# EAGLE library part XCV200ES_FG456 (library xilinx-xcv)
xcv200es_fg456 edit this description Auto generated by make-symbol-device-package-bsdl.ulp Rev. 26 Source: xcv200es_fg456.bsd
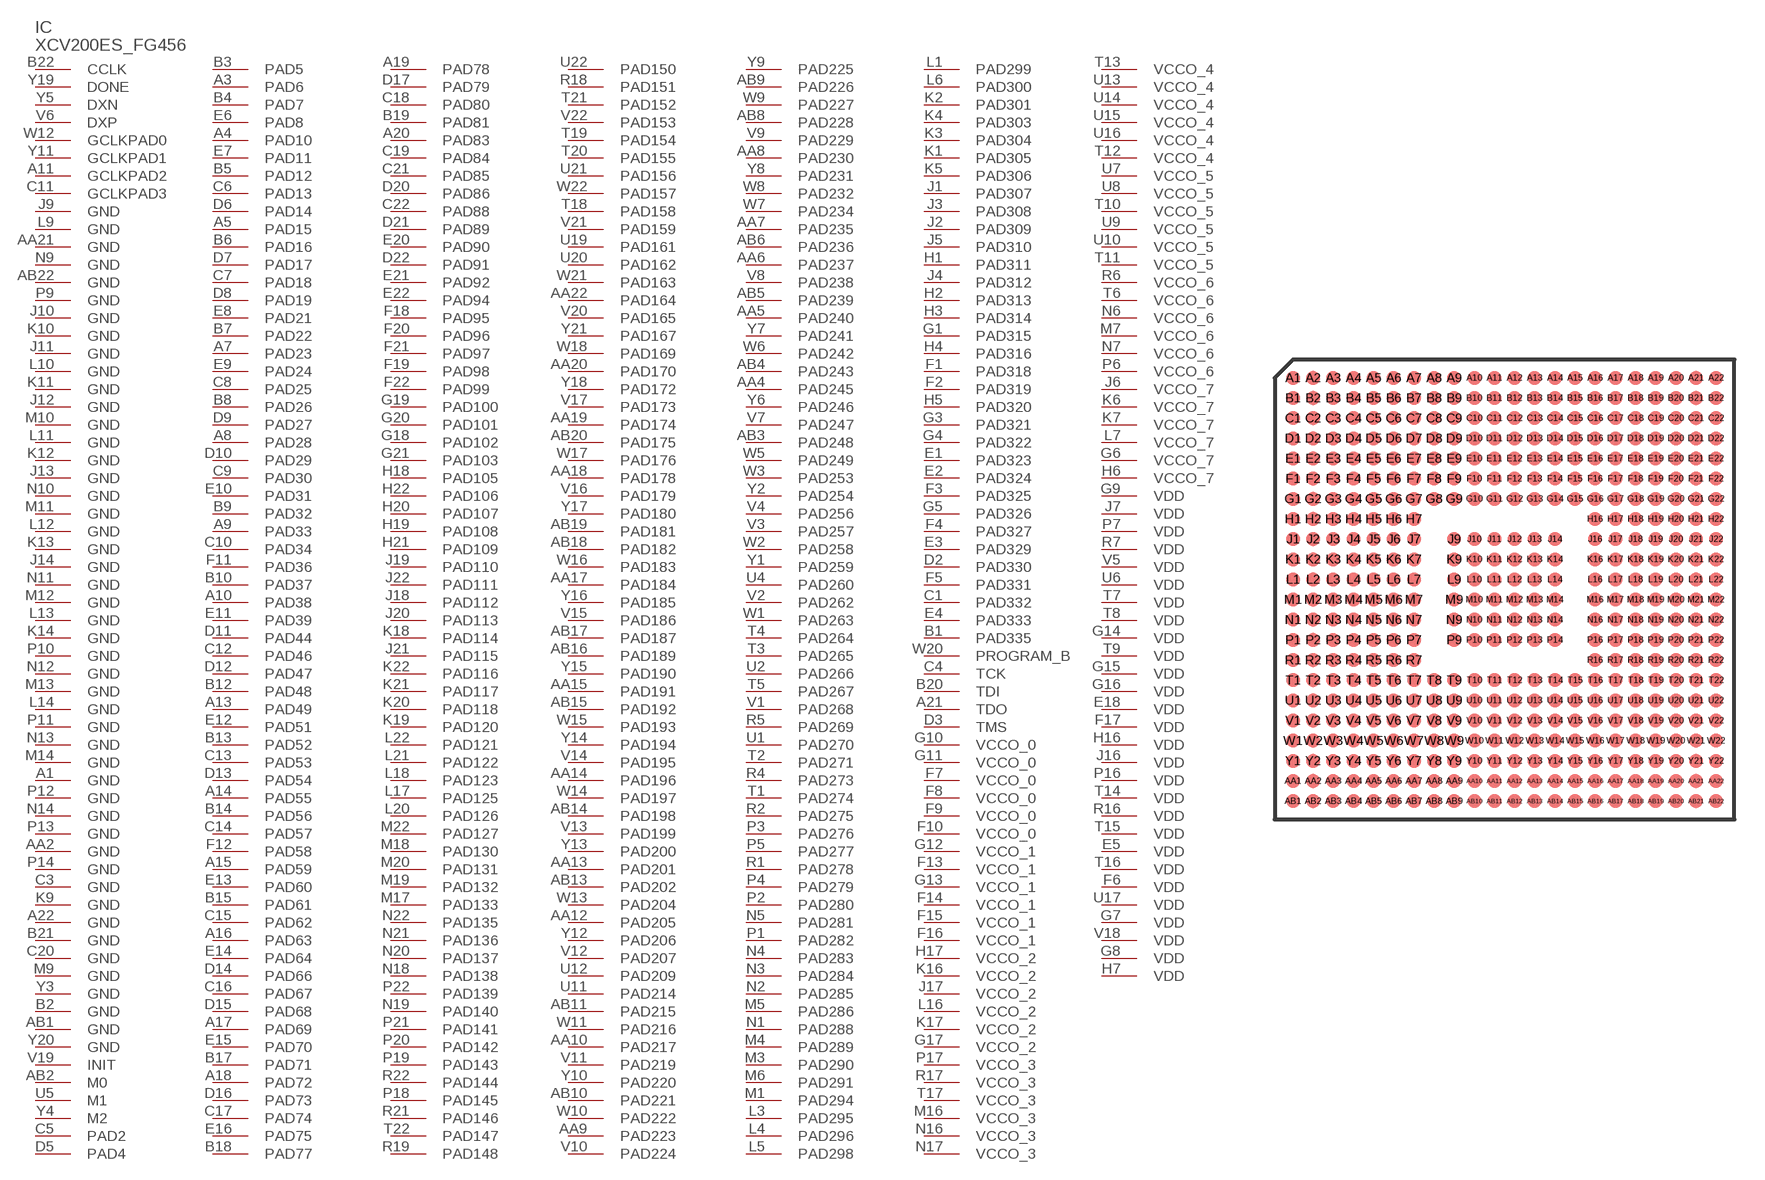
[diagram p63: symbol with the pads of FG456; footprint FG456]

Designator prefix IC

## XCV200ES_FG456 (OC_FARNELL: unknown; OC_NEWARK: unknown)  [FG456]
A1  GND  pwr
A3  PAD6
A4  PAD10
A5  PAD15
A7  PAD23
A8  PAD28
A9  PAD33
A10  PAD38
A11  GCLKPAD2  in
A13  PAD49
A14  PAD55
A15  PAD59
A16  PAD63
A17  PAD69
A18  PAD72
A19  PAD78
A20  PAD83
A21  TDO  out
A22  GND  pwr
AA2  GND  pwr
AA4  PAD245
AA5  PAD240
AA6  PAD237
AA7  PAD235
AA8  PAD230
AA9  PAD223
AA10  PAD217
AA12  PAD205
AA13  PAD201
AA14  PAD196
AA15  PAD191
AA17  PAD184
AA18  PAD178
AA19  PAD174
AA20  PAD170
AA21  GND  pwr
AA22  PAD164
AB1  GND  pwr
AB2  M0  in
AB3  PAD248
AB4  PAD243
AB5  PAD239
AB6  PAD236
AB8  PAD228
AB9  PAD226
AB10  PAD221
AB11  PAD215
AB13  PAD202
AB14  PAD198
AB15  PAD192
AB16  PAD189
AB17  PAD187
AB18  PAD182
AB19  PAD181
AB20  PAD175
AB22  GND  pwr
B1  PAD335
B2  GND  pwr
B3  PAD5
B4  PAD7
B5  PAD12
B6  PAD16
B7  PAD22
B8  PAD26
B9  PAD32
B10  PAD37
B12  PAD48
B13  PAD52
B14  PAD56
B15  PAD61
B17  PAD71
B18  PAD77
B19  PAD81
B20  TDI  in
B21  GND  pwr
B22  CCLK
C1  PAD332
C3  GND  pwr
C4  TCK  in
C5  PAD2
C6  PAD13
C7  PAD18
C8  PAD25
C9  PAD30
C10  PAD34
C11  GCLKPAD3  in
C12  PAD46
C13  PAD53
C14  PAD57
C15  PAD62
C16  PAD67
C17  PAD74
C18  PAD80
C19  PAD84
C20  GND  pwr
C21  PAD85
C22  PAD88
D2  PAD330
D3  TMS  in
D5  PAD4
D6  PAD14
D7  PAD17
D8  PAD19
D9  PAD27
D10  PAD29
D11  PAD44
D12  PAD47
D13  PAD54
D14  PAD66
D15  PAD68
D16  PAD73
D17  PAD79
D20  PAD86
D21  PAD89
D22  PAD91
E1  PAD323
E2  PAD324
E3  PAD329
E4  PAD333
E5  VDD  pwr
E6  PAD8
E7  PAD11
E8  PAD21
E9  PAD24
E10  PAD31
E11  PAD39
E12  PAD51
E13  PAD60
E14  PAD64
E15  PAD70
E16  PAD75
E18  VDD  pwr
E20  PAD90
E21  PAD92
E22  PAD94
F1  PAD318
F2  PAD319
F3  PAD325
F4  PAD327
F5  PAD331
F6  VDD  pwr
F7  VCCO_0  pwr
F8  VCCO_0  pwr
F9  VCCO_0  pwr
F10  VCCO_0  pwr
F11  PAD36
F12  PAD58
F13  VCCO_1  pwr
F14  VCCO_1  pwr
F15  VCCO_1  pwr
F16  VCCO_1  pwr
F17  VDD  pwr
F18  PAD95
F19  PAD98
F20  PAD96
F21  PAD97
F22  PAD99
G1  PAD315
G3  PAD321
G4  PAD322
G5  PAD326
G6  VCCO_7  pwr
G7  VDD  pwr
G8  VDD  pwr
G9  VDD  pwr
G10  VCCO_0  pwr
G11  VCCO_0  pwr
G12  VCCO_1  pwr
G13  VCCO_1  pwr
G14  VDD  pwr
G15  VDD  pwr
G16  VDD  pwr
G17  VCCO_2  pwr
G18  PAD102
G19  PAD100
G20  PAD101
G21  PAD103
H1  PAD311
H2  PAD313
H3  PAD314
H4  PAD316
H5  PAD320
H6  VCCO_7  pwr
H7  VDD  pwr
H16  VDD  pwr
H17  VCCO_2  pwr
H18  PAD105
H19  PAD108
H20  PAD107
H21  PAD109
H22  PAD106
J1  PAD307
J2  PAD309
J3  PAD308
J4  PAD312
J5  PAD310
J6  VCCO_7  pwr
J7  VDD  pwr
J9  GND  pwr
J10  GND  pwr
J11  GND  pwr
J12  GND  pwr
J13  GND  pwr
J14  GND  pwr
J16  VDD  pwr
J17  VCCO_2  pwr
J18  PAD112
J19  PAD110
J20  PAD113
J21  PAD115
J22  PAD111
K1  PAD305
K2  PAD301
K3  PAD304
K4  PAD303
K5  PAD306
K6  VCCO_7  pwr
K7  VCCO_7  pwr
K9  GND  pwr
K10  GND  pwr
K11  GND  pwr
K12  GND  pwr
K13  GND  pwr
K14  GND  pwr
K16  VCCO_2  pwr
K17  VCCO_2  pwr
K18  PAD114
K19  PAD120
K20  PAD118
K21  PAD117
K22  PAD116
L1  PAD299
L3  PAD295
L4  PAD296
L5  PAD298
L6  PAD300
L7  VCCO_7  pwr
L9  GND  pwr
L10  GND  pwr
L11  GND  pwr
L12  GND  pwr
L13  GND  pwr
L14  GND  pwr
L16  VCCO_2  pwr
L17  PAD125
L18  PAD123
L20  PAD126
L21  PAD122
L22  PAD121
M1  PAD294
M3  PAD290
M4  PAD289
M5  PAD286
M6  PAD291
M7  VCCO_6  pwr
M9  GND  pwr
M10  GND  pwr
M11  GND  pwr
M12  GND  pwr
M13  GND  pwr
M14  GND  pwr
M16  VCCO_3  pwr
M17  PAD133
M18  PAD130
M19  PAD132
M20  PAD131
M22  PAD127
N1  PAD288
N2  PAD285
N3  PAD284
N4  PAD283
N5  PAD281
N6  VCCO_6  pwr
N7  VCCO_6  pwr
N9  GND  pwr
N10  GND  pwr
N11  GND  pwr
N12  GND  pwr
N13  GND  pwr
N14  GND  pwr
N16  VCCO_3  pwr
N17  VCCO_3  pwr
N18  PAD138
N19  PAD140
N20  PAD137
N21  PAD136
N22  PAD135
P1  PAD282
P2  PAD280
P3  PAD276
P4  PAD279
P5  PAD277
P6  VCCO_6  pwr
P7  VDD  pwr
P9  GND  pwr
P10  GND  pwr
P11  GND  pwr
P12  GND  pwr
P13  GND  pwr
P14  GND  pwr
P16  VDD  pwr
P17  VCCO_3  pwr
P18  PAD145
P19  PAD143
P20  PAD142
P21  PAD141
P22  PAD139
R1  PAD278
R2  PAD275
R4  PAD273
R5  PAD269
R6  VCCO_6  pwr
R7  VDD  pwr
R16  VDD  pwr
R17  VCCO_3  pwr
R18  PAD151
R19  PAD148
R21  PAD146
R22  PAD144
T1  PAD274
T2  PAD271
T3  PAD265
T4  PAD264
T5  PAD267
T6  VCCO_6  pwr
T7  VDD  pwr
T8  VDD  pwr
T9  VDD  pwr
T10  VCCO_5  pwr
T11  VCCO_5  pwr
T12  VCCO_4  pwr
T13  VCCO_4  pwr
T14  VDD  pwr
T15  VDD  pwr
T16  VDD  pwr
T17  VCCO_3  pwr
T18  PAD158
T19  PAD154
T20  PAD155
T21  PAD152
T22  PAD147
U1  PAD270
U2  PAD266
U4  PAD260
U5  M1  in
U6  VDD  pwr
U7  VCCO_5  pwr
U8  VCCO_5  pwr
U9  VCCO_5  pwr
U10  VCCO_5  pwr
U11  PAD214
U12  PAD209
U13  VCCO_4  pwr
U14  VCCO_4  pwr
U15  VCCO_4  pwr
U16  VCCO_4  pwr
U17  VDD  pwr
U19  PAD161
U20  PAD162
U21  PAD156
U22  PAD150
V1  PAD268
V2  PAD262
V3  PAD257
V4  PAD256
V5  VDD  pwr
V6  DXP  pas
V7  PAD247
V8  PAD238
V9  PAD229
V10  PAD224
V11  PAD219
V12  PAD207
V13  PAD199
V14  PAD195
V15  PAD186
V16  PAD179
V17  PAD173
V18  VDD  pwr
V19  INIT
V20  PAD165
V21  PAD159
V22  PAD153
W1  PAD263
W2  PAD258
W3  PAD253
W5  PAD249
W6  PAD242
W7  PAD234
W8  PAD232
W9  PAD227
W10  PAD222
W11  PAD216
W12  GCLKPAD0  in
W13  PAD204
W14  PAD197
W15  PAD193
W16  PAD183
W17  PAD176
W18  PAD169
W20  PROGRAM_B  in
W21  PAD163
W22  PAD157
Y1  PAD259
Y2  PAD254
Y3  GND  pwr
Y4  M2  in
Y5  DXN  pas
Y6  PAD246
Y7  PAD241
Y8  PAD231
Y9  PAD225
Y10  PAD220
Y11  GCLKPAD1  in
Y12  PAD206
Y13  PAD200
Y14  PAD194
Y15  PAD190
Y16  PAD185
Y17  PAD180
Y18  PAD172
Y19  DONE
Y20  GND  pwr
Y21  PAD167

## Footprint FG456 (pad centres in mm)
xcv150_fg456 edit this description Auto generated by make-symbol-device-package-bsdl.ulp Rev. 26 Source: xcv150_fg456.bsd
smd 0.7 x 0.7: A1 -10.5,10.5; A2 -9.5,10.5; A3 -8.5,10.5; A4 -7.5,10.5; A5 -6.5,10.5; A6 -5.5,10.5; A7 -4.5,10.5; A8 -3.5,10.5; A9 -2.5,10.5; A10 -1.5,10.5; A11 -0.5,10.5; A12 0.5,10.5; A13 1.5,10.5; A14 2.5,10.5; A15 3.5,10.5; A16 4.5,10.5; A17 5.5,10.5; A18 6.5,10.5; A19 7.5,10.5; A20 8.5,10.5; A21 9.5,10.5; A22 10.5,10.5; AA1 -10.5,-9.5; AA2 -9.5,-9.5; AA3 -8.5,-9.5; AA4 -7.5,-9.5; AA5 -6.5,-9.5; AA6 -5.5,-9.5; AA7 -4.5,-9.5; AA8 -3.5,-9.5; AA9 -2.5,-9.5; AA10 -1.5,-9.5; AA11 -0.5,-9.5; AA12 0.5,-9.5; AA13 1.5,-9.5; AA14 2.5,-9.5; AA15 3.5,-9.5; AA16 4.5,-9.5; AA17 5.5,-9.5; AA18 6.5,-9.5; AA19 7.5,-9.5; AA20 8.5,-9.5; AA21 9.5,-9.5; AA22 10.5,-9.5; AB1 -10.5,-10.5; AB2 -9.5,-10.5; AB3 -8.5,-10.5; AB4 -7.5,-10.5; AB5 -6.5,-10.5; AB6 -5.5,-10.5; AB7 -4.5,-10.5; AB8 -3.5,-10.5; AB9 -2.5,-10.5; AB10 -1.5,-10.5; AB11 -0.5,-10.5; AB12 0.5,-10.5; AB13 1.5,-10.5; AB14 2.5,-10.5; AB15 3.5,-10.5; AB16 4.5,-10.5; AB17 5.5,-10.5; AB18 6.5,-10.5; AB19 7.5,-10.5; AB20 8.5,-10.5; AB21 9.5,-10.5; AB22 10.5,-10.5; B1 -10.5,9.5; B2 -9.5,9.5; B3 -8.5,9.5; B4 -7.5,9.5; B5 -6.5,9.5; B6 -5.5,9.5; B7 -4.5,9.5; B8 -3.5,9.5; B9 -2.5,9.5; B10 -1.5,9.5; B11 -0.5,9.5; B12 0.5,9.5; B13 1.5,9.5; B14 2.5,9.5; B15 3.5,9.5; B16 4.5,9.5; B17 5.5,9.5; B18 6.5,9.5; B19 7.5,9.5; B20 8.5,9.5; B21 9.5,9.5; B22 10.5,9.5; C1 -10.5,8.5; C2 -9.5,8.5; C3 -8.5,8.5; C4 -7.5,8.5; C5 -6.5,8.5; C6 -5.5,8.5; C7 -4.5,8.5; C8 -3.5,8.5; C9 -2.5,8.5; C10 -1.5,8.5; C11 -0.5,8.5; C12 0.5,8.5; C13 1.5,8.5; C14 2.5,8.5; C15 3.5,8.5; C16 4.5,8.5; C17 5.5,8.5; C18 6.5,8.5; C19 7.5,8.5; C20 8.5,8.5; C21 9.5,8.5; C22 10.5,8.5; D1 -10.5,7.5; D2 -9.5,7.5; D3 -8.5,7.5; D4 -7.5,7.5; D5 -6.5,7.5; D6 -5.5,7.5; D7 -4.5,7.5; D8 -3.5,7.5; D9 -2.5,7.5; D10 -1.5,7.5; D11 -0.5,7.5; D12 0.5,7.5; D13 1.5,7.5; D14 2.5,7.5; D15 3.5,7.5; D16 4.5,7.5; D17 5.5,7.5; D18 6.5,7.5; D19 7.5,7.5; D20 8.5,7.5; D21 9.5,7.5; D22 10.5,7.5; E1 -10.5,6.5; E2 -9.5,6.5; E3 -8.5,6.5; E4 -7.5,6.5; E5 -6.5,6.5; E6 -5.5,6.5; E7 -4.5,6.5; E8 -3.5,6.5; E9 -2.5,6.5; E10 -1.5,6.5; E11 -0.5,6.5; E12 0.5,6.5; E13 1.5,6.5; E14 2.5,6.5; E15 3.5,6.5; E16 4.5,6.5; E17 5.5,6.5; E18 6.5,6.5; E19 7.5,6.5; E20 8.5,6.5; E21 9.5,6.5; E22 10.5,6.5; F1 -10.5,5.5; F2 -9.5,5.5; F3 -8.5,5.5; F4 -7.5,5.5; F5 -6.5,5.5; F6 -5.5,5.5; F7 -4.5,5.5; F8 -3.5,5.5; F9 -2.5,5.5; F10 -1.5,5.5; F11 -0.5,5.5; F12 0.5,5.5; F13 1.5,5.5; F14 2.5,5.5; F15 3.5,5.5; F16 4.5,5.5; F17 5.5,5.5; F18 6.5,5.5; F19 7.5,5.5; F20 8.5,5.5; F21 9.5,5.5; F22 10.5,5.5; G1 -10.5,4.5; G2 -9.5,4.5; G3 -8.5,4.5; G4 -7.5,4.5; G5 -6.5,4.5; G6 -5.5,4.5; G7 -4.5,4.5; G8 -3.5,4.5; G9 -2.5,4.5; G10 -1.5,4.5; G11 -0.5,4.5; G12 0.5,4.5; G13 1.5,4.5; G14 2.5,4.5; G15 3.5,4.5; G16 4.5,4.5; G17 5.5,4.5; G18 6.5,4.5; G19 7.5,4.5; G20 8.5,4.5; G21 9.5,4.5; G22 10.5,4.5; H1 -10.5,3.5; H2 -9.5,3.5; H3 -8.5,3.5; H4 -7.5,3.5; H5 -6.5,3.5; H6 -5.5,3.5; H7 -4.5,3.5; H16 4.5,3.5; H17 5.5,3.5; H18 6.5,3.5; H19 7.5,3.5; H20 8.5,3.5; H21 9.5,3.5; H22 10.5,3.5; J1 -10.5,2.5; J2 -9.5,2.5; J3 -8.5,2.5; J4 -7.5,2.5; J5 -6.5,2.5; J6 -5.5,2.5; J7 -4.5,2.5; J9 -2.5,2.5; J10 -1.5,2.5; J11 -0.5,2.5; J12 0.5,2.5; J13 1.5,2.5; J14 2.5,2.5; J16 4.5,2.5; J17 5.5,2.5; J18 6.5,2.5; J19 7.5,2.5; J20 8.5,2.5; J21 9.5,2.5; J22 10.5,2.5; K1 -10.5,1.5; K2 -9.5,1.5; K3 -8.5,1.5; K4 -7.5,1.5; K5 -6.5,1.5; K6 -5.5,1.5; K7 -4.5,1.5; K9 -2.5,1.5; K10 -1.5,1.5; K11 -0.5,1.5; K12 0.5,1.5; K13 1.5,1.5; K14 2.5,1.5; K16 4.5,1.5; K17 5.5,1.5; K18 6.5,1.5; K19 7.5,1.5; K20 8.5,1.5; K21 9.5,1.5; K22 10.5,1.5; L1 -10.5,0.5; L2 -9.5,0.5; L3 -8.5,0.5; L4 -7.5,0.5; L5 -6.5,0.5; L6 -5.5,0.5; L7 -4.5,0.5; L9 -2.5,0.5; L10 -1.5,0.5; L11 -0.5,0.5; L12 0.5,0.5; L13 1.5,0.5; L14 2.5,0.5; L16 4.5,0.5; L17 5.5,0.5; L18 6.5,0.5; L19 7.5,0.5; L20 8.5,0.5; L21 9.5,0.5; L22 10.5,0.5; M1 -10.5,-0.5; M2 -9.5,-0.5; M3 -8.5,-0.5; M4 -7.5,-0.5; M5 -6.5,-0.5; M6 -5.5,-0.5; M7 -4.5,-0.5; M9 -2.5,-0.5; M10 -1.5,-0.5; M11 -0.5,-0.5; M12 0.5,-0.5; M13 1.5,-0.5; M14 2.5,-0.5; M16 4.5,-0.5; M17 5.5,-0.5; M18 6.5,-0.5; M19 7.5,-0.5; M20 8.5,-0.5; M21 9.5,-0.5; M22 10.5,-0.5; N1 -10.5,-1.5; N2 -9.5,-1.5; N3 -8.5,-1.5; N4 -7.5,-1.5; N5 -6.5,-1.5; N6 -5.5,-1.5; N7 -4.5,-1.5; N9 -2.5,-1.5; N10 -1.5,-1.5; N11 -0.5,-1.5; N12 0.5,-1.5; N13 1.5,-1.5; N14 2.5,-1.5; N16 4.5,-1.5; N17 5.5,-1.5; N18 6.5,-1.5; N19 7.5,-1.5; N20 8.5,-1.5; N21 9.5,-1.5; N22 10.5,-1.5; P1 -10.5,-2.5; P2 -9.5,-2.5; P3 -8.5,-2.5; P4 -7.5,-2.5; P5 -6.5,-2.5; P6 -5.5,-2.5; P7 -4.5,-2.5; P9 -2.5,-2.5; P10 -1.5,-2.5; P11 -0.5,-2.5; P12 0.5,-2.5; P13 1.5,-2.5; P14 2.5,-2.5; P16 4.5,-2.5; P17 5.5,-2.5; P18 6.5,-2.5; P19 7.5,-2.5; P20 8.5,-2.5; P21 9.5,-2.5; P22 10.5,-2.5; R1 -10.5,-3.5; R2 -9.5,-3.5; R3 -8.5,-3.5; R4 -7.5,-3.5; R5 -6.5,-3.5; R6 -5.5,-3.5; R7 -4.5,-3.5; R16 4.5,-3.5; R17 5.5,-3.5; R18 6.5,-3.5; R19 7.5,-3.5; R20 8.5,-3.5; R21 9.5,-3.5; R22 10.5,-3.5; T1 -10.5,-4.5; T2 -9.5,-4.5; T3 -8.5,-4.5; T4 -7.5,-4.5; T5 -6.5,-4.5; T6 -5.5,-4.5; T7 -4.5,-4.5; T8 -3.5,-4.5; T9 -2.5,-4.5; T10 -1.5,-4.5; T11 -0.5,-4.5; T12 0.5,-4.5; T13 1.5,-4.5; T14 2.5,-4.5; T15 3.5,-4.5; T16 4.5,-4.5; T17 5.5,-4.5; T18 6.5,-4.5; T19 7.5,-4.5; T20 8.5,-4.5; T21 9.5,-4.5; T22 10.5,-4.5; U1 -10.5,-5.5; U2 -9.5,-5.5; U3 -8.5,-5.5; U4 -7.5,-5.5; U5 -6.5,-5.5; U6 -5.5,-5.5; U7 -4.5,-5.5; U8 -3.5,-5.5; U9 -2.5,-5.5; U10 -1.5,-5.5; U11 -0.5,-5.5; U12 0.5,-5.5; U13 1.5,-5.5; U14 2.5,-5.5; U15 3.5,-5.5; U16 4.5,-5.5; U17 5.5,-5.5; U18 6.5,-5.5; U19 7.5,-5.5; U20 8.5,-5.5; U21 9.5,-5.5; U22 10.5,-5.5; V1 -10.5,-6.5; V2 -9.5,-6.5; V3 -8.5,-6.5; V4 -7.5,-6.5; V5 -6.5,-6.5; V6 -5.5,-6.5; V7 -4.5,-6.5; V8 -3.5,-6.5; V9 -2.5,-6.5; V10 -1.5,-6.5; V11 -0.5,-6.5; V12 0.5,-6.5; V13 1.5,-6.5; V14 2.5,-6.5; V15 3.5,-6.5; V16 4.5,-6.5; V17 5.5,-6.5; V18 6.5,-6.5; V19 7.5,-6.5; V20 8.5,-6.5; V21 9.5,-6.5; V22 10.5,-6.5; W1 -10.5,-7.5; W2 -9.5,-7.5; W3 -8.5,-7.5; W4 -7.5,-7.5; W5 -6.5,-7.5; W6 -5.5,-7.5; W7 -4.5,-7.5; W8 -3.5,-7.5; W9 -2.5,-7.5; W10 -1.5,-7.5; W11 -0.5,-7.5; W12 0.5,-7.5; W13 1.5,-7.5; W14 2.5,-7.5; W15 3.5,-7.5; W16 4.5,-7.5; W17 5.5,-7.5; W18 6.5,-7.5; W19 7.5,-7.5; W20 8.5,-7.5; W21 9.5,-7.5; W22 10.5,-7.5; Y1 -10.5,-8.5; Y2 -9.5,-8.5; Y3 -8.5,-8.5; Y4 -7.5,-8.5; Y5 -6.5,-8.5; Y6 -5.5,-8.5; Y7 -4.5,-8.5; Y8 -3.5,-8.5; Y9 -2.5,-8.5; Y10 -1.5,-8.5; Y11 -0.5,-8.5; Y12 0.5,-8.5; Y13 1.5,-8.5; Y14 2.5,-8.5; Y15 3.5,-8.5; Y16 4.5,-8.5; Y17 5.5,-8.5; Y18 6.5,-8.5; Y19 7.5,-8.5; Y20 8.5,-8.5; Y21 9.5,-8.5; Y22 10.5,-8.5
